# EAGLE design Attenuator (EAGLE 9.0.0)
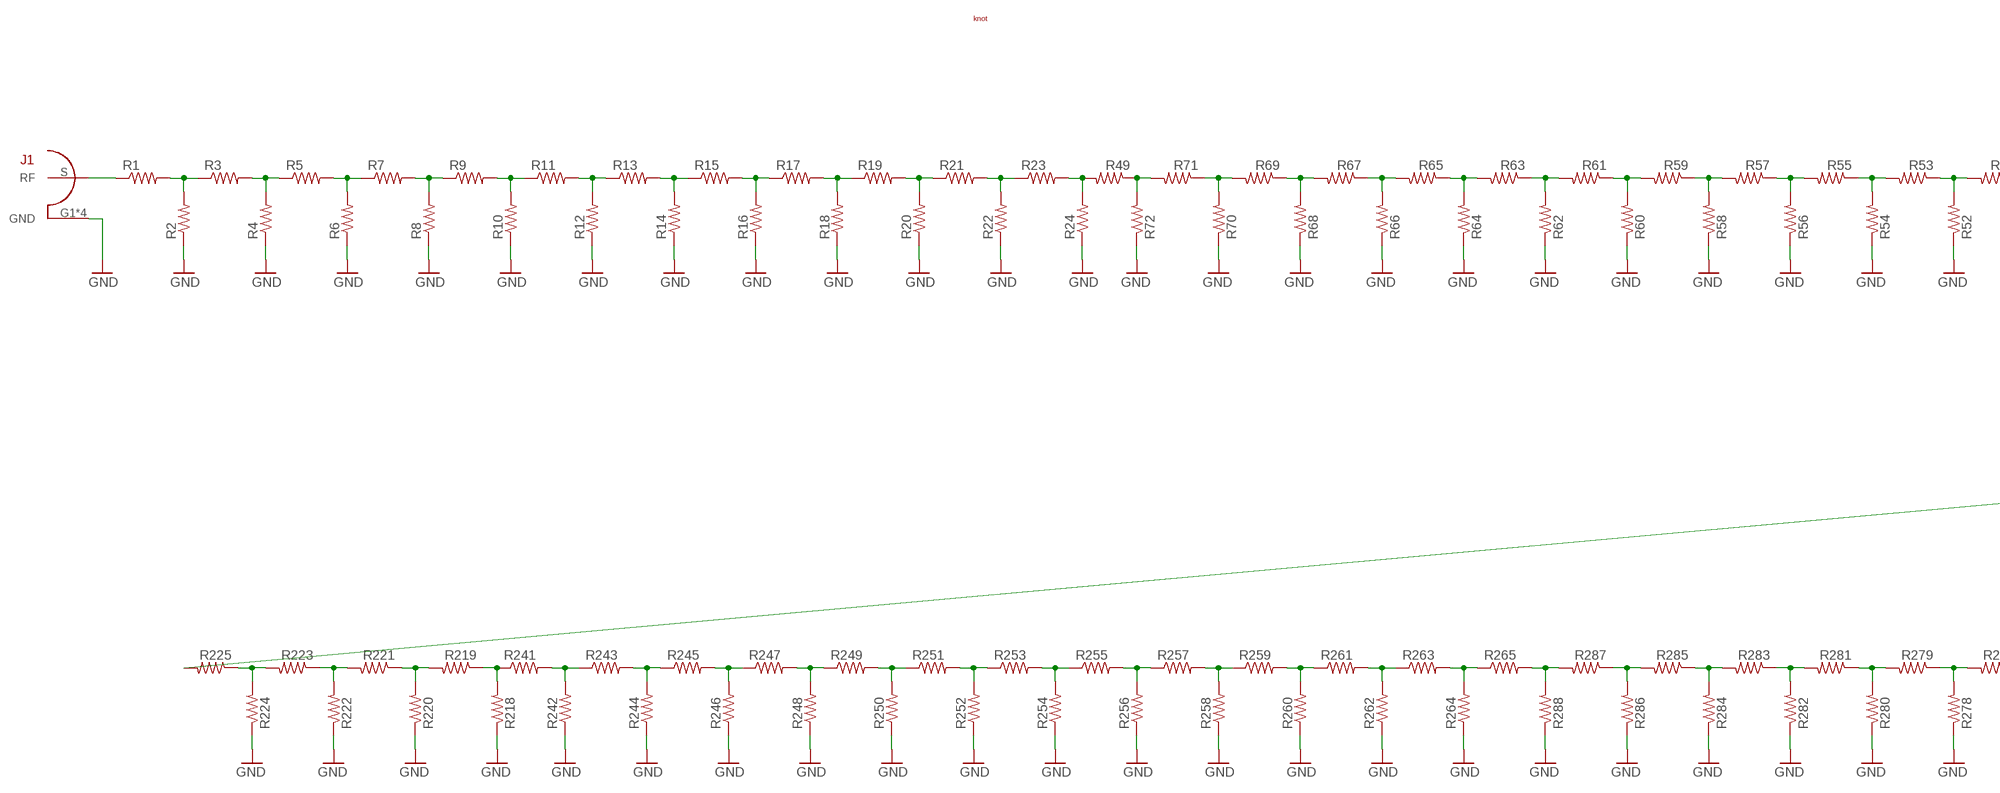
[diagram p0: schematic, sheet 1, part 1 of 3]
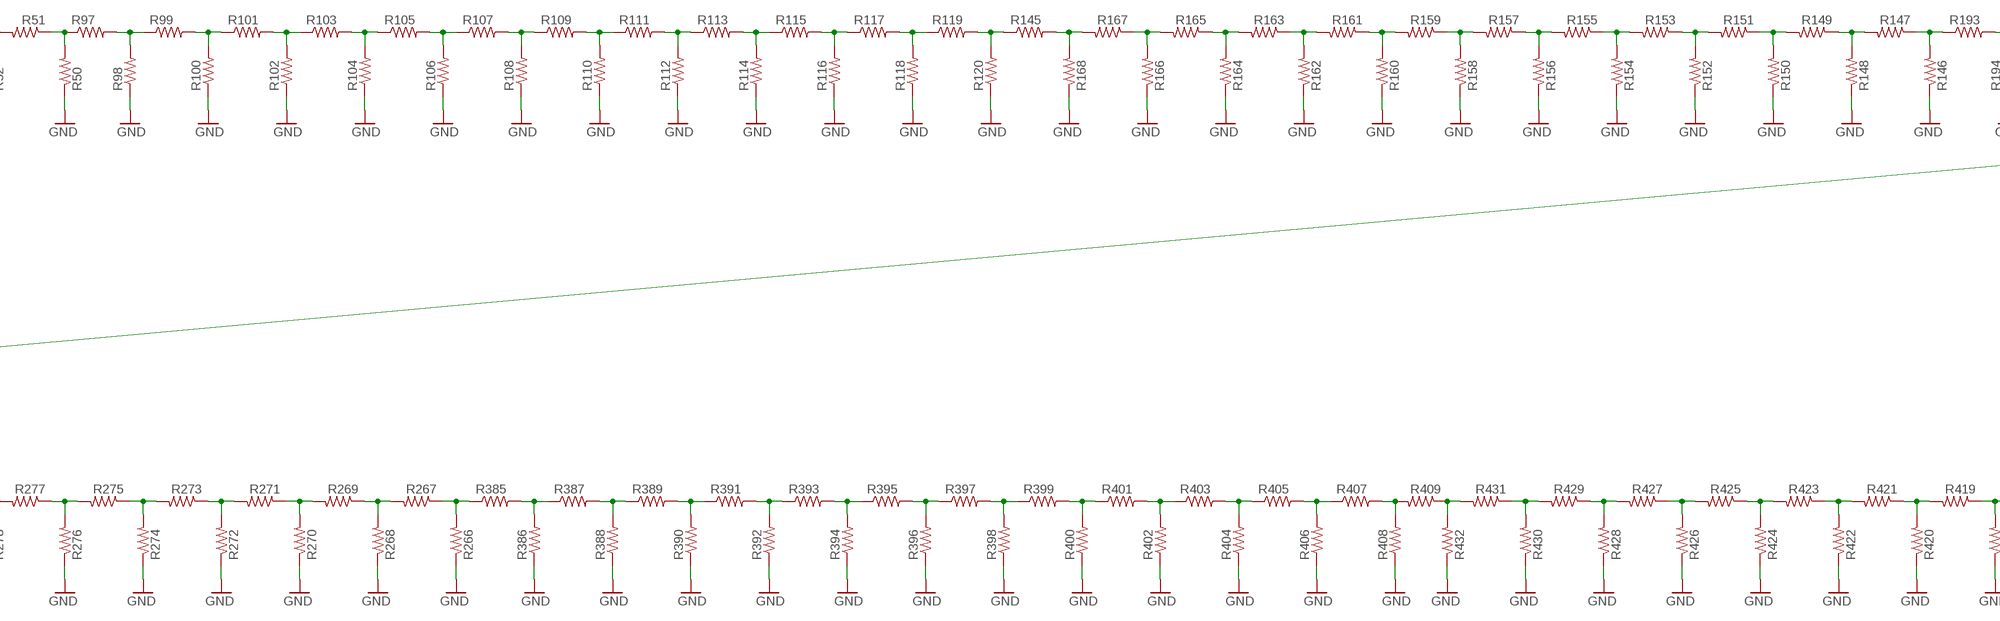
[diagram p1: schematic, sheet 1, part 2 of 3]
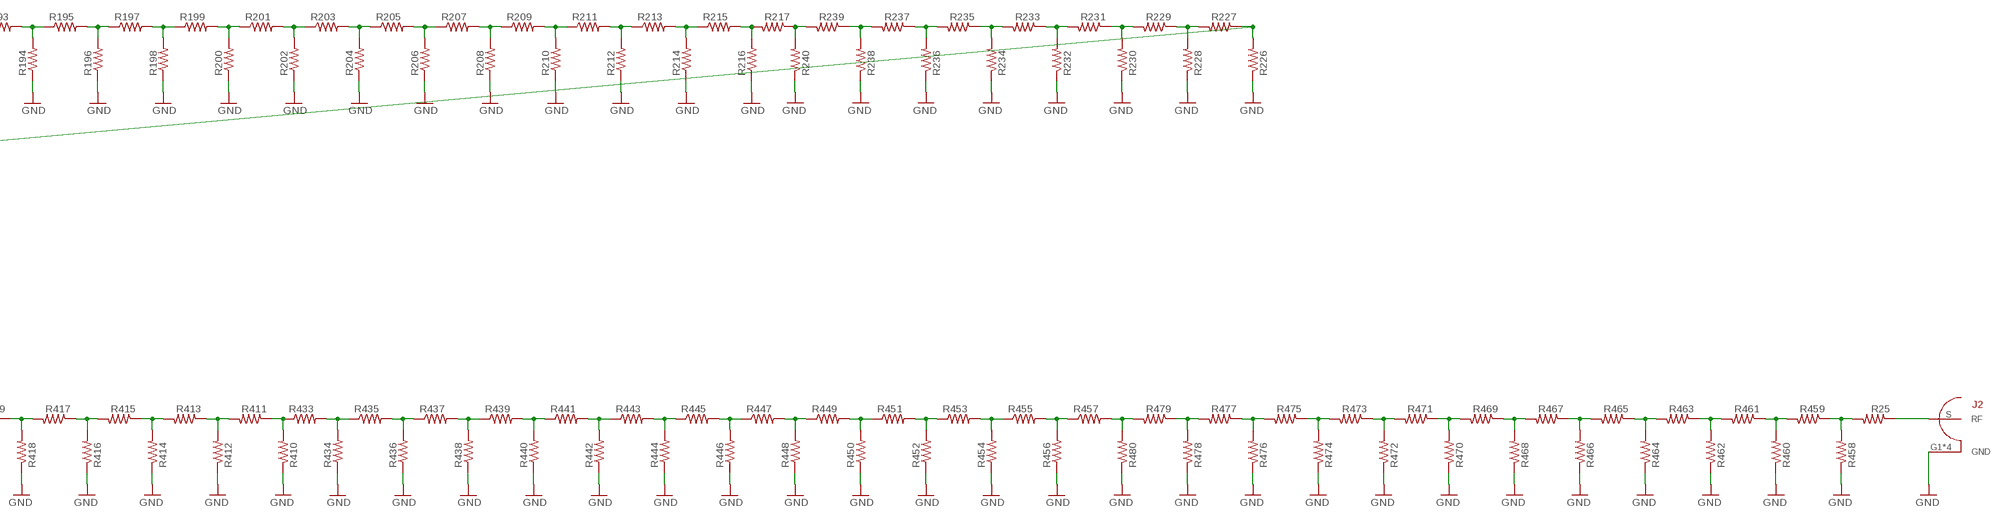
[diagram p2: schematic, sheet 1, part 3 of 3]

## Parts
J1  SMA_0732511150  [WIDE_SMA]
J2  SMA_0732511150  [WIDE_SMA]
R1  R-US_R1206  [R1206]
R2  R-US_R1206  [R1206]
R3  R-US_R1206  [R1206]
R4  R-US_R1206  [R1206]
R5  R-US_R1206  [R1206]
R6  R-US_R1206  [R1206]
R7  R-US_R1206  [R1206]
R8  R-US_R1206  [R1206]
R9  R-US_R1206  [R1206]
R10  R-US_R1206  [R1206]
R11  R-US_R1206  [R1206]
R12  R-US_R1206  [R1206]
R13  R-US_R1206  [R1206]
R14  R-US_R1206  [R1206]
R15  R-US_R1206  [R1206]
R16  R-US_R1206  [R1206]
R17  R-US_R1206  [R1206]
R18  R-US_R1206  [R1206]
R19  R-US_R1206  [R1206]
R20  R-US_R1206  [R1206]
R21  R-US_R1206  [R1206]
R22  R-US_R1206  [R1206]
R23  R-US_R1206  [R1206]
R24  R-US_R1206  [R1206]
R25  R-US_R1206  [R1206]
R49  R-US_R1206  [R1206]
R50  R-US_R1206  [R1206]
R51  R-US_R1206  [R1206]
R52  R-US_R1206  [R1206]
R53  R-US_R1206  [R1206]
R54  R-US_R1206  [R1206]
R55  R-US_R1206  [R1206]
R56  R-US_R1206  [R1206]
R57  R-US_R1206  [R1206]
R58  R-US_R1206  [R1206]
R59  R-US_R1206  [R1206]
R60  R-US_R1206  [R1206]
R61  R-US_R1206  [R1206]
R62  R-US_R1206  [R1206]
R63  R-US_R1206  [R1206]
R64  R-US_R1206  [R1206]
R65  R-US_R1206  [R1206]
R66  R-US_R1206  [R1206]
R67  R-US_R1206  [R1206]
R68  R-US_R1206  [R1206]
R69  R-US_R1206  [R1206]
R70  R-US_R1206  [R1206]
R71  R-US_R1206  [R1206]
R72  R-US_R1206  [R1206]
R97  R-US_R1206  [R1206]
R98  R-US_R1206  [R1206]
R99  R-US_R1206  [R1206]
R100  R-US_R1206  [R1206]
R101  R-US_R1206  [R1206]
R102  R-US_R1206  [R1206]
R103  R-US_R1206  [R1206]
R104  R-US_R1206  [R1206]
R105  R-US_R1206  [R1206]
R106  R-US_R1206  [R1206]
R107  R-US_R1206  [R1206]
R108  R-US_R1206  [R1206]
R109  R-US_R1206  [R1206]
R110  R-US_R1206  [R1206]
R111  R-US_R1206  [R1206]
R112  R-US_R1206  [R1206]
R113  R-US_R1206  [R1206]
R114  R-US_R1206  [R1206]
R115  R-US_R1206  [R1206]
R116  R-US_R1206  [R1206]
R117  R-US_R1206  [R1206]
R118  R-US_R1206  [R1206]
R119  R-US_R1206  [R1206]
R120  R-US_R1206  [R1206]
R145  R-US_R1206  [R1206]
R146  R-US_R1206  [R1206]
R147  R-US_R1206  [R1206]
R148  R-US_R1206  [R1206]
R149  R-US_R1206  [R1206]
R150  R-US_R1206  [R1206]
R151  R-US_R1206  [R1206]
R152  R-US_R1206  [R1206]
R153  R-US_R1206  [R1206]
R154  R-US_R1206  [R1206]
R155  R-US_R1206  [R1206]
R156  R-US_R1206  [R1206]
R157  R-US_R1206  [R1206]
R158  R-US_R1206  [R1206]
R159  R-US_R1206  [R1206]
R160  R-US_R1206  [R1206]
R161  R-US_R1206  [R1206]
R162  R-US_R1206  [R1206]
R163  R-US_R1206  [R1206]
R164  R-US_R1206  [R1206]
R165  R-US_R1206  [R1206]
R166  R-US_R1206  [R1206]
R167  R-US_R1206  [R1206]
R168  R-US_R1206  [R1206]
R193  R-US_R1206  [R1206]
R194  R-US_R1206  [R1206]
R195  R-US_R1206  [R1206]
R196  R-US_R1206  [R1206]
R197  R-US_R1206  [R1206]
R198  R-US_R1206  [R1206]
R199  R-US_R1206  [R1206]
R200  R-US_R1206  [R1206]
R201  R-US_R1206  [R1206]
R202  R-US_R1206  [R1206]
R203  R-US_R1206  [R1206]
R204  R-US_R1206  [R1206]
R205  R-US_R1206  [R1206]
R206  R-US_R1206  [R1206]
R207  R-US_R1206  [R1206]
R208  R-US_R1206  [R1206]
R209  R-US_R1206  [R1206]
R210  R-US_R1206  [R1206]
R211  R-US_R1206  [R1206]
R212  R-US_R1206  [R1206]
R213  R-US_R1206  [R1206]
R214  R-US_R1206  [R1206]
R215  R-US_R1206  [R1206]
R216  R-US_R1206  [R1206]
R217  R-US_R1206  [R1206]
R218  R-US_R1206  [R1206]
R219  R-US_R1206  [R1206]
R220  R-US_R1206  [R1206]
R221  R-US_R1206  [R1206]
R222  R-US_R1206  [R1206]
R223  R-US_R1206  [R1206]
R224  R-US_R1206  [R1206]
R225  R-US_R1206  [R1206]
R226  R-US_R1206  [R1206]
R227  R-US_R1206  [R1206]
R228  R-US_R1206  [R1206]
R229  R-US_R1206  [R1206]
R230  R-US_R1206  [R1206]
R231  R-US_R1206  [R1206]
R232  R-US_R1206  [R1206]
R233  R-US_R1206  [R1206]
R234  R-US_R1206  [R1206]
R235  R-US_R1206  [R1206]
R236  R-US_R1206  [R1206]
R237  R-US_R1206  [R1206]
R238  R-US_R1206  [R1206]
R239  R-US_R1206  [R1206]
R240  R-US_R1206  [R1206]
R241  R-US_R1206  [R1206]
R242  R-US_R1206  [R1206]
R243  R-US_R1206  [R1206]
R244  R-US_R1206  [R1206]
R245  R-US_R1206  [R1206]
R246  R-US_R1206  [R1206]
R247  R-US_R1206  [R1206]
R248  R-US_R1206  [R1206]
R249  R-US_R1206  [R1206]
R250  R-US_R1206  [R1206]
R251  R-US_R1206  [R1206]
R252  R-US_R1206  [R1206]
R253  R-US_R1206  [R1206]
R254  R-US_R1206  [R1206]
R255  R-US_R1206  [R1206]
R256  R-US_R1206  [R1206]
R257  R-US_R1206  [R1206]
R258  R-US_R1206  [R1206]
R259  R-US_R1206  [R1206]
R260  R-US_R1206  [R1206]
R261  R-US_R1206  [R1206]
R262  R-US_R1206  [R1206]
R263  R-US_R1206  [R1206]
R264  R-US_R1206  [R1206]
R265  R-US_R1206  [R1206]
R266  R-US_R1206  [R1206]
R267  R-US_R1206  [R1206]
R268  R-US_R1206  [R1206]
R269  R-US_R1206  [R1206]
R270  R-US_R1206  [R1206]
R271  R-US_R1206  [R1206]
R272  R-US_R1206  [R1206]
R273  R-US_R1206  [R1206]
R274  R-US_R1206  [R1206]
R275  R-US_R1206  [R1206]
R276  R-US_R1206  [R1206]
R277  R-US_R1206  [R1206]
R278  R-US_R1206  [R1206]
R279  R-US_R1206  [R1206]
R280  R-US_R1206  [R1206]
R281  R-US_R1206  [R1206]
R282  R-US_R1206  [R1206]
R283  R-US_R1206  [R1206]
R284  R-US_R1206  [R1206]
R285  R-US_R1206  [R1206]
R286  R-US_R1206  [R1206]
R287  R-US_R1206  [R1206]
R288  R-US_R1206  [R1206]
R385  R-US_R1206  [R1206]
R386  R-US_R1206  [R1206]
R387  R-US_R1206  [R1206]
R388  R-US_R1206  [R1206]
R389  R-US_R1206  [R1206]
R390  R-US_R1206  [R1206]
R391  R-US_R1206  [R1206]
R392  R-US_R1206  [R1206]
R393  R-US_R1206  [R1206]
R394  R-US_R1206  [R1206]
R395  R-US_R1206  [R1206]
R396  R-US_R1206  [R1206]
R397  R-US_R1206  [R1206]
R398  R-US_R1206  [R1206]
R399  R-US_R1206  [R1206]
R400  R-US_R1206  [R1206]
R401  R-US_R1206  [R1206]
R402  R-US_R1206  [R1206]
R403  R-US_R1206  [R1206]
R404  R-US_R1206  [R1206]
R405  R-US_R1206  [R1206]
R406  R-US_R1206  [R1206]
R407  R-US_R1206  [R1206]
R408  R-US_R1206  [R1206]
R409  R-US_R1206  [R1206]
R410  R-US_R1206  [R1206]
R411  R-US_R1206  [R1206]
R412  R-US_R1206  [R1206]
R413  R-US_R1206  [R1206]
R414  R-US_R1206  [R1206]
R415  R-US_R1206  [R1206]
R416  R-US_R1206  [R1206]
R417  R-US_R1206  [R1206]
R418  R-US_R1206  [R1206]
R419  R-US_R1206  [R1206]
R420  R-US_R1206  [R1206]
R421  R-US_R1206  [R1206]
R422  R-US_R1206  [R1206]
R423  R-US_R1206  [R1206]
R424  R-US_R1206  [R1206]
R425  R-US_R1206  [R1206]
R426  R-US_R1206  [R1206]
R427  R-US_R1206  [R1206]
R428  R-US_R1206  [R1206]
R429  R-US_R1206  [R1206]
R430  R-US_R1206  [R1206]
R431  R-US_R1206  [R1206]
R432  R-US_R1206  [R1206]
R433  R-US_R1206  [R1206]
R434  R-US_R1206  [R1206]
R435  R-US_R1206  [R1206]
R436  R-US_R1206  [R1206]
R437  R-US_R1206  [R1206]
R438  R-US_R1206  [R1206]
R439  R-US_R1206  [R1206]
R440  R-US_R1206  [R1206]
R441  R-US_R1206  [R1206]
R442  R-US_R1206  [R1206]
R443  R-US_R1206  [R1206]
R444  R-US_R1206  [R1206]
R445  R-US_R1206  [R1206]
R446  R-US_R1206  [R1206]
R447  R-US_R1206  [R1206]
R448  R-US_R1206  [R1206]
R449  R-US_R1206  [R1206]
R450  R-US_R1206  [R1206]
R451  R-US_R1206  [R1206]
R452  R-US_R1206  [R1206]
R453  R-US_R1206  [R1206]
R454  R-US_R1206  [R1206]
R455  R-US_R1206  [R1206]
R456  R-US_R1206  [R1206]
R457  R-US_R1206  [R1206]
R458  R-US_R1206  [R1206]
R459  R-US_R1206  [R1206]
R460  R-US_R1206  [R1206]
R461  R-US_R1206  [R1206]
R462  R-US_R1206  [R1206]
R463  R-US_R1206  [R1206]
R464  R-US_R1206  [R1206]
R465  R-US_R1206  [R1206]
R466  R-US_R1206  [R1206]
R467  R-US_R1206  [R1206]
R468  R-US_R1206  [R1206]
R469  R-US_R1206  [R1206]
R470  R-US_R1206  [R1206]
R471  R-US_R1206  [R1206]
R472  R-US_R1206  [R1206]
R473  R-US_R1206  [R1206]
R474  R-US_R1206  [R1206]
R475  R-US_R1206  [R1206]
R476  R-US_R1206  [R1206]
R477  R-US_R1206  [R1206]
R478  R-US_R1206  [R1206]
R479  R-US_R1206  [R1206]
R480  R-US_R1206  [R1206]
U$1  THIEF_FULL  [THIEF_KNOT]

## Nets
GND: J1.G1(GND) J1.G2(GND) J1.G3(GND) J1.G4(GND) J2.G1(GND) J2.G2(GND) J2.G3(GND) J2.G4(GND) R2.1 R4.1 R6.1 R8.1 R10.1 R12.1 R14.1 R16.1 R18.1 R20.1 R22.1 R24.1 R50.1 R52.1 R54.1 R56.1 R58.1 R60.1 R62.1 R64.1 R66.1 R68.1 R70.1 R72.1 R98.1 R100.1 R102.1 R104.1 R106.1 R108.1 R110.1 R112.1 R114.1 R116.1 R118.1 R120.1 R146.1 R148.1 R150.1 R152.1 R154.1 R156.1 R158.1 R160.1 R162.1 R164.1 R166.1 R168.1 R194.1 R196.1 R198.1 R200.1 R202.1 R204.1 R206.1 R208.1 R210.1 R212.1 R214.1 R216.1 R218.1 R220.1 R222.1 R224.1 R226.1 R228.1 R230.1 R232.1 R234.1 R236.1 R238.1 R240.1 R242.1 R244.1 R246.1 R248.1 R250.1 R252.1 R254.1 R256.1 R258.1 R260.1 R262.1 R264.1 R266.1 R268.1 R270.1 R272.1 R274.1 R276.1 R278.1 R280.1 R282.1 R284.1 R286.1 R288.1 R386.1 R388.1 R390.1 R392.1 R394.1 R396.1 R398.1 R400.1 R402.1 R404.1 R406.1 R408.1 R410.1 R412.1 R414.1 R416.1 R418.1 R420.1 R422.1 R424.1 R426.1 R428.1 R430.1 R432.1 R434.1 R436.1 R438.1 R440.1 R442.1 R444.1 R446.1 R448.1 R450.1 R452.1 R454.1 R456.1 R458.1 R460.1 R462.1 R464.1 R466.1 R468.1 R470.1 R472.1 R474.1 R476.1 R478.1 R480.1
N$1: R1.2 R2.2 R3.1
N$2: R3.2 R4.2 R5.1
N$3: R5.2 R6.2 R7.1
N$4: R7.2 R8.2 R9.1
N$5: R9.2 R10.2 R11.1
N$6: R11.2 R12.2 R13.1
N$7: R13.2 R14.2 R15.1
N$8: R15.2 R16.2 R17.1
N$9: R17.2 R18.2 R19.1
N$10: R19.2 R20.2 R21.1
N$11: R21.2 R22.2 R23.1
N$12: R23.2 R24.2 R49.2
N$13: J1.S(RF) R1.1
N$14: J2.S(RF) R25.1
N$25: R50.2 R51.1 R97.1
N$26: R51.2 R52.2 R53.1
N$27: R53.2 R54.2 R55.1
N$28: R55.2 R56.2 R57.1
N$29: R57.2 R58.2 R59.1
N$30: R59.2 R60.2 R61.1
N$31: R61.2 R62.2 R63.1
N$32: R63.2 R64.2 R65.1
N$33: R65.2 R66.2 R67.1
N$34: R67.2 R68.2 R69.1
N$35: R69.2 R70.2 R71.1
N$36: R49.1 R71.2 R72.2
N$49: R97.2 R98.2 R99.1
N$50: R99.2 R100.2 R101.1
N$51: R101.2 R102.2 R103.1
N$52: R103.2 R104.2 R105.1
N$53: R105.2 R106.2 R107.1
N$54: R107.2 R108.2 R109.1
N$55: R109.2 R110.2 R111.1
N$56: R111.2 R112.2 R113.1
N$57: R113.2 R114.2 R115.1
N$58: R115.2 R116.2 R117.1
N$59: R117.2 R118.2 R119.1
N$60: R119.2 R120.2 R145.1
N$73: R146.2 R147.1 R193.1
N$74: R147.2 R148.2 R149.1
N$75: R149.2 R150.2 R151.1
N$76: R151.2 R152.2 R153.1
N$77: R153.2 R154.2 R155.1
N$78: R155.2 R156.2 R157.1
N$79: R157.2 R158.2 R159.1
N$80: R159.2 R160.2 R161.1
N$81: R161.2 R162.2 R163.1
N$82: R163.2 R164.2 R165.1
N$83: R165.2 R166.2 R167.1
N$84: R145.2 R167.2 R168.2
N$97: R193.2 R194.2 R195.1
N$98: R195.2 R196.2 R197.1
N$99: R197.2 R198.2 R199.1
N$100: R199.2 R200.2 R201.1
N$101: R201.2 R202.2 R203.1
N$102: R203.2 R204.2 R205.1
N$103: R205.2 R206.2 R207.1
N$104: R207.2 R208.2 R209.1
N$105: R209.2 R210.2 R211.1
N$106: R211.2 R212.2 R213.1
N$107: R213.2 R214.2 R215.1
N$108: R215.2 R216.2 R217.2
N$109: R218.2 R219.1 R241.1
N$110: R219.2 R220.2 R221.1
N$111: R221.2 R222.2 R223.1
N$112: R223.2 R224.2 R225.1
N$113: R225.2 R226.2 R227.1
N$114: R227.2 R228.2 R229.1
N$115: R229.2 R230.2 R231.1
N$116: R231.2 R232.2 R233.1
N$117: R233.2 R234.2 R235.1
N$118: R235.2 R236.2 R237.1
N$119: R237.2 R238.2 R239.1
N$120: R217.1 R239.2 R240.2
N$121: R241.2 R242.2 R243.1
N$122: R243.2 R244.2 R245.1
N$123: R245.2 R246.2 R247.1
N$124: R247.2 R248.2 R249.1
N$125: R249.2 R250.2 R251.1
N$126: R251.2 R252.2 R253.1
N$127: R253.2 R254.2 R255.1
N$128: R255.2 R256.2 R257.1
N$129: R257.2 R258.2 R259.1
N$130: R259.2 R260.2 R261.1
N$131: R261.2 R262.2 R263.1
N$132: R263.2 R264.2 R265.1
N$133: R266.2 R267.1 R385.1
N$134: R267.2 R268.2 R269.1
N$135: R269.2 R270.2 R271.1
N$136: R271.2 R272.2 R273.1
N$137: R273.2 R274.2 R275.1
N$138: R275.2 R276.2 R277.1
N$139: R277.2 R278.2 R279.1
N$140: R279.2 R280.2 R281.1
N$141: R281.2 R282.2 R283.1
N$142: R283.2 R284.2 R285.1
N$143: R285.2 R286.2 R287.1
N$144: R265.2 R287.2 R288.2
N$193: R385.2 R386.2 R387.1
N$194: R387.2 R388.2 R389.1
N$195: R389.2 R390.2 R391.1
N$196: R391.2 R392.2 R393.1
N$197: R393.2 R394.2 R395.1
N$198: R395.2 R396.2 R397.1
N$199: R397.2 R398.2 R399.1
N$200: R399.2 R400.2 R401.1
N$201: R401.2 R402.2 R403.1
N$202: R403.2 R404.2 R405.1
N$203: R405.2 R406.2 R407.1
N$204: R407.2 R408.2 R409.2
N$205: R410.2 R411.1 R433.1
N$206: R411.2 R412.2 R413.1
N$207: R413.2 R414.2 R415.1
N$208: R415.2 R416.2 R417.1
N$209: R417.2 R418.2 R419.1
N$210: R419.2 R420.2 R421.1
N$211: R421.2 R422.2 R423.1
N$212: R423.2 R424.2 R425.1
N$213: R425.2 R426.2 R427.1
N$214: R427.2 R428.2 R429.1
N$215: R429.2 R430.2 R431.1
N$216: R409.1 R431.2 R432.2
N$217: R433.2 R434.2 R435.1
N$218: R435.2 R436.2 R437.1
N$219: R437.2 R438.2 R439.1
N$220: R439.2 R440.2 R441.1
N$221: R441.2 R442.2 R443.1
N$222: R443.2 R444.2 R445.1
N$223: R445.2 R446.2 R447.1
N$224: R447.2 R448.2 R449.1
N$225: R449.2 R450.2 R451.1
N$226: R451.2 R452.2 R453.1
N$227: R453.2 R454.2 R455.1
N$228: R455.2 R456.2 R457.1
N$229: R25.2 R458.2 R459.1
N$230: R459.2 R460.2 R461.1
N$231: R461.2 R462.2 R463.1
N$232: R463.2 R464.2 R465.1
N$233: R465.2 R466.2 R467.1
N$234: R467.2 R468.2 R469.1
N$235: R469.2 R470.2 R471.1
N$236: R471.2 R472.2 R473.1
N$237: R473.2 R474.2 R475.1
N$238: R475.2 R476.2 R477.1
N$239: R477.2 R478.2 R479.1
N$240: R457.2 R479.2 R480.2

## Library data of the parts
J1 J2 = ruark2:SMA_0732511150: SMA Connector Receptacle, Female Socket 50 Ohm Board Edge, End Launch Solder; PARTNO: WM5534-ND
R1-R25 R49-R72 R97-R120 R145-R168 R193-R288 R385-R480 = resistor:R-US_: RESISTOR, American symbol
U$1 = ruark2:THIEF_FULL; PARTNO: NA

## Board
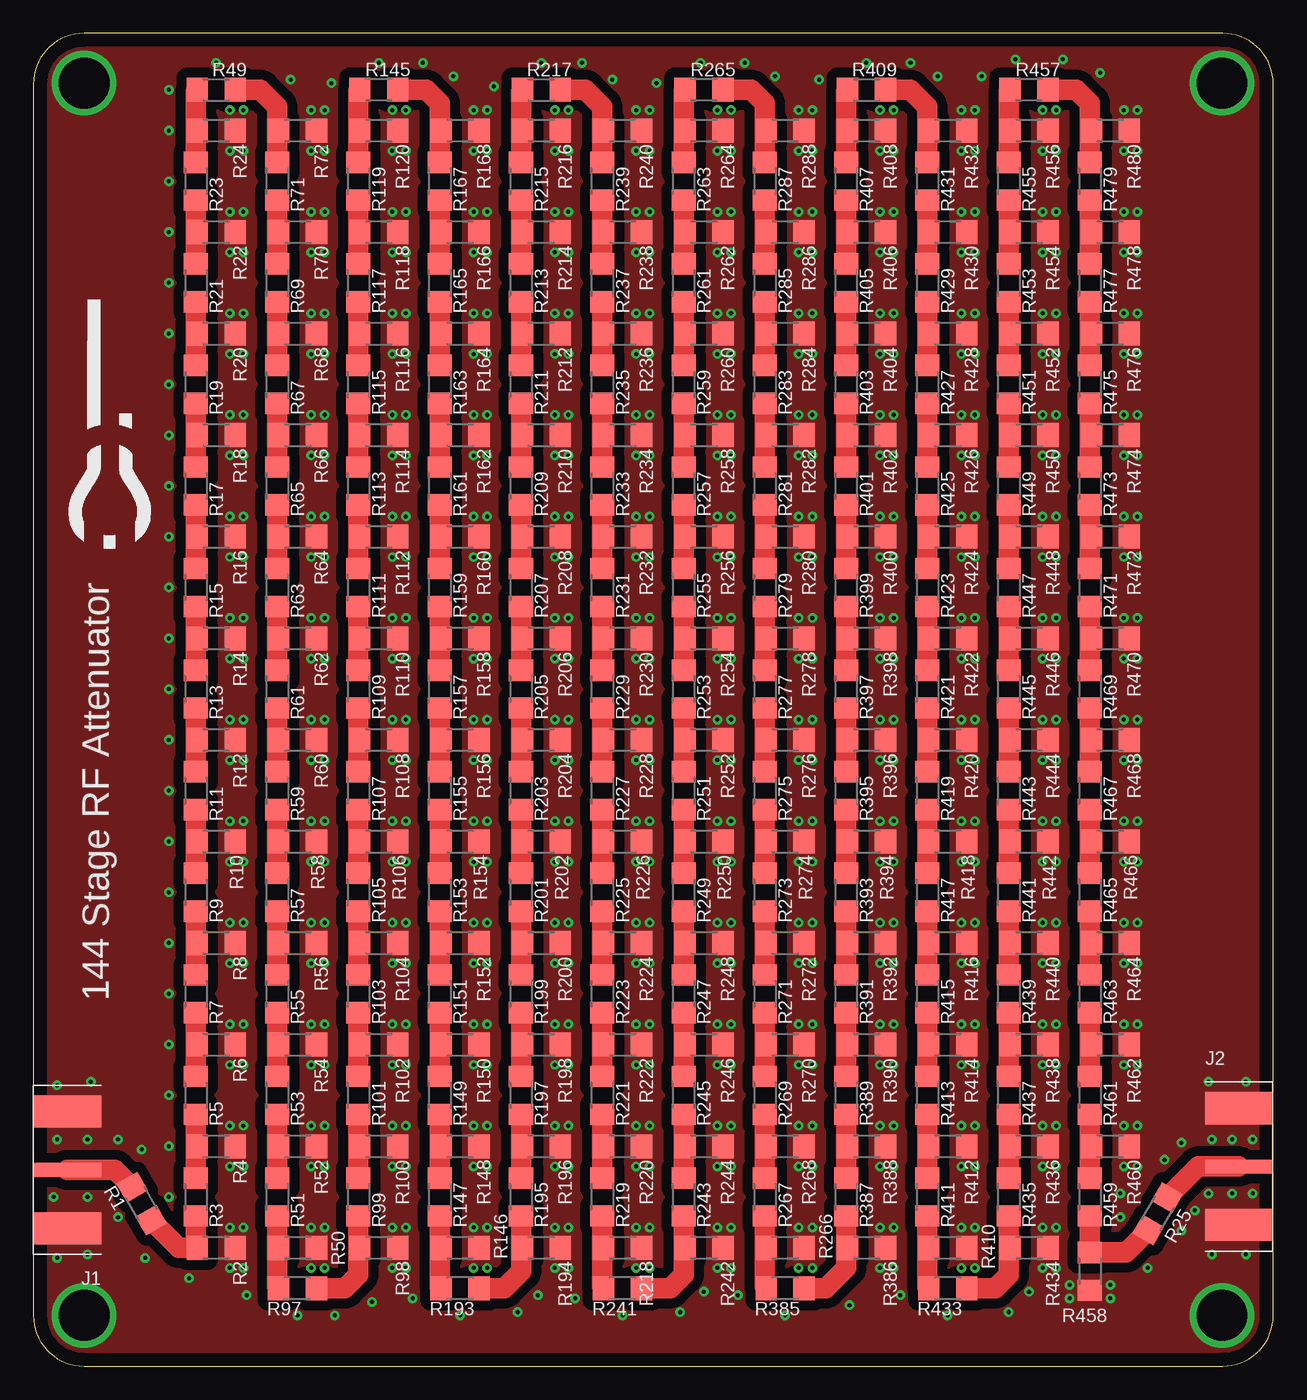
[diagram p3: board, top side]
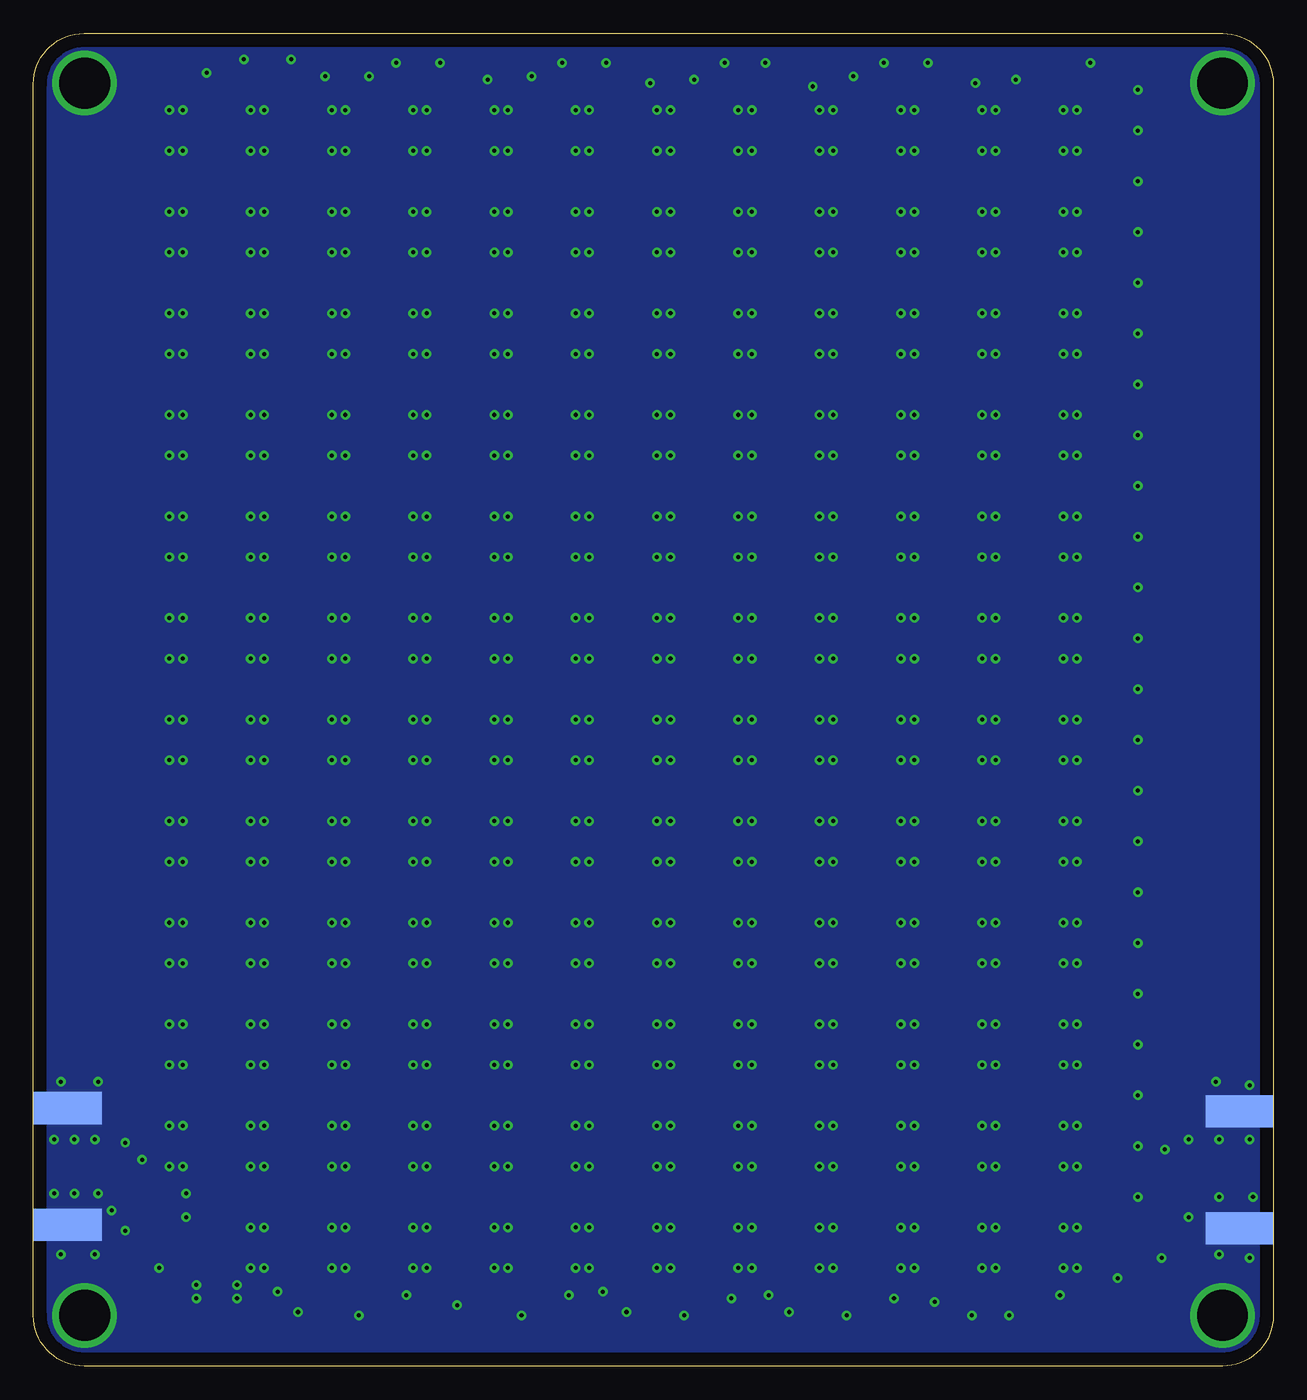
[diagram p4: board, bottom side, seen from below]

Size 93 x 100 mm. Coordinates in mm from the lower left corner, seen from the top.
Outline: 3.81,0 89.19,0 arc90 93,3.81 93,96.19 arc90 89.19,100 3.81,100 arc90 0,96.19 0,3.81 arc90 3.81,0
Copper layers (1*16): Top 0.035mm / dielectric 1.5mm / Bottom 0.035mm
Design rules "default": minimum track width 6mil, minimum drill 0.35mm, track to track 6mil, track to pad 6mil, pad to pad 6mil, via to via 6mil, smd to smd 6mil, copper to edge 40mil, drill to drill 6mil, minimum pad ring 10mil, minimum via ring 8mil, stop-mask expansion 4mil, vias tented up to drill 0mil, thermal gap 10mil

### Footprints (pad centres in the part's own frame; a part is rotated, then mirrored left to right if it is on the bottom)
WIDE_SMA = smd 5.08 x 2.413 bottom: G1 0,4.381; G4 0,-4.381 | smd 5.08 x 2.413: G2 0,-4.381; G3 0,4.381 | smd 5.08 x 1.016: S 0,0
R1206 = smd 1.6 x 1.803: 1 -1.422,0; 2 1.422,0

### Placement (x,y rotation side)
J1  2.54,14.73 180 top
J2  90.42,14.99 0 top
R1  8.13,12.19 300 top
R2  13.72,8.89 180 top
R3  12.19,12.7 90 top
R4  13.72,16.51 180 top
R5  12.19,20.32 90 top
R6  13.72,24.13 180 top
R7  12.19,27.94 90 top
R8  13.72,31.75 180 top
R9  12.19,35.56 90 top
R10  13.72,39.37 180 top
R11  12.19,43.18 90 top
R12  13.72,46.99 180 top
R13  12.19,50.8 90 top
R14  13.72,54.61 180 top
R15  12.19,58.42 90 top
R16  13.72,62.23 180 top
R17  12.19,66.04 90 top
R18  13.72,69.85 180 top
R19  12.19,73.66 90 top
R20  13.72,77.47 180 top
R21  12.19,81.28 90 top
R22  13.72,85.09 180 top
R23  12.19,88.9 90 top
R24  13.72,92.71 180 top
R25  84.33,11.43 240 top
R49  13.72,95.76 180 top
R50  19.81,8.89 180 top
R51  18.29,12.7 90 top
R52  19.81,16.51 180 top
R53  18.29,20.32 90 top
R54  19.81,24.13 180 top
R55  18.29,27.94 90 top
R56  19.81,31.75 180 top
R57  18.29,35.56 90 top
R58  19.81,39.37 180 top
R59  18.29,43.18 90 top
R60  19.81,46.99 180 top
R61  18.29,50.8 90 top
R62  19.81,54.61 180 top
R63  18.29,58.42 90 top
R64  19.81,62.23 180 top
R65  18.29,66.04 90 top
R66  19.81,69.85 180 top
R67  18.29,73.66 90 top
R68  19.81,77.47 180 top
R69  18.29,81.28 90 top
R70  19.81,85.09 180 top
R71  18.29,88.9 90 top
R72  19.81,92.71 180 top
R97  19.81,5.84 0 top
R98  25.91,8.89 180 top
R99  24.38,12.7 90 top
R100  25.91,16.51 180 top
R101  24.38,20.32 90 top
R102  25.91,24.13 180 top
R103  24.38,27.94 90 top
R104  25.91,31.75 180 top
R105  24.38,35.56 90 top
R106  25.91,39.37 180 top
R107  24.38,43.18 90 top
R108  25.91,46.99 180 top
R109  24.38,50.8 90 top
R110  25.91,54.61 180 top
R111  24.38,58.42 90 top
R112  25.91,62.23 180 top
R113  24.38,66.04 90 top
R114  25.91,69.85 180 top
R115  24.38,73.66 90 top
R116  25.91,77.47 180 top
R117  24.38,81.28 90 top
R118  25.91,85.09 180 top
R119  24.38,88.9 90 top
R120  25.91,92.71 180 top
R145  25.91,95.76 0 top
R146  32,8.89 180 top
R147  30.48,12.7 90 top
R148  32,16.51 180 top
R149  30.48,20.32 90 top
R150  32,24.13 180 top
R151  30.48,27.94 90 top
R152  32,31.75 180 top
R153  30.48,35.56 90 top
R154  32,39.37 180 top
R155  30.48,43.18 90 top
R156  32,46.99 180 top
R157  30.48,50.8 90 top
R158  32,54.61 180 top
R159  30.48,58.42 90 top
R160  32,62.23 180 top
R161  30.48,66.04 90 top
R162  32,69.85 180 top
R163  30.48,73.66 90 top
R164  32,77.47 180 top
R165  30.48,81.28 90 top
R166  32,85.09 180 top
R167  30.48,88.9 90 top
R168  32,92.71 180 top
R193  32,5.84 0 top
R194  38.1,8.89 180 top
R195  36.58,12.7 90 top
R196  38.1,16.51 180 top
R197  36.58,20.32 90 top
R198  38.1,24.13 180 top
R199  36.58,27.94 90 top
R200  38.1,31.75 180 top
R201  36.58,35.56 90 top
R202  38.1,39.37 180 top
R203  36.58,43.18 90 top
R204  38.1,46.99 180 top
R205  36.58,50.8 90 top
R206  38.1,54.61 180 top
R207  36.58,58.42 90 top
R208  38.1,62.23 180 top
R209  36.58,66.04 90 top
R210  38.1,69.85 180 top
R211  36.58,73.66 90 top
R212  38.1,77.47 180 top
R213  36.58,81.28 90 top
R214  38.1,85.09 180 top
R215  36.58,88.9 90 top
R216  38.1,92.71 180 top
R217  38.1,95.76 180 top
R218  44.2,8.89 180 top
R219  42.67,12.7 90 top
R220  44.2,16.51 180 top
R221  42.67,20.32 90 top
R222  44.2,24.13 180 top
R223  42.67,27.94 90 top
R224  44.2,31.75 180 top
R225  42.67,35.56 90 top
R226  44.2,39.37 180 top
R227  42.67,43.18 90 top
R228  44.2,46.99 180 top
R229  42.67,50.8 90 top
R230  44.2,54.61 180 top
R231  42.67,58.42 90 top
R232  44.2,62.23 180 top
R233  42.67,66.04 90 top
R234  44.2,69.85 180 top
R235  42.67,73.66 90 top
R236  44.2,77.47 180 top
R237  42.67,81.28 90 top
R238  44.2,85.09 180 top
R239  42.67,88.9 90 top
R240  44.2,92.71 180 top
R241  44.2,5.84 0 top
R242  50.29,8.89 180 top
R243  48.77,12.7 90 top
R244  50.29,16.51 180 top
R245  48.77,20.32 90 top
R246  50.29,24.13 180 top
R247  48.77,27.94 90 top
R248  50.29,31.75 180 top
R249  48.77,35.56 90 top
R250  50.29,39.37 180 top
R251  48.77,43.18 90 top
R252  50.29,46.99 180 top
R253  48.77,50.8 90 top
R254  50.29,54.61 180 top
R255  48.77,58.42 90 top
R256  50.29,62.23 180 top
R257  48.77,66.04 90 top
R258  50.29,69.85 180 top
R259  48.77,73.66 90 top
R260  50.29,77.47 180 top
R261  48.77,81.28 90 top
R262  50.29,85.09 180 top
R263  48.77,88.9 90 top
R264  50.29,92.71 180 top
R265  50.29,95.76 0 top
R266  56.39,8.89 180 top
R267  54.86,12.7 90 top
R268  56.39,16.51 180 top
R269  54.86,20.32 90 top
R270  56.39,24.13 180 top
R271  54.86,27.94 90 top
R272  56.39,31.75 180 top
R273  54.86,35.56 90 top
R274  56.39,39.37 180 top
R275  54.86,43.18 90 top
R276  56.39,46.99 180 top
R277  54.86,50.8 90 top
R278  56.39,54.61 180 top
R279  54.86,58.42 90 top
R280  56.39,62.23 180 top
R281  54.86,66.04 90 top
R282  56.39,69.85 180 top
R283  54.86,73.66 90 top
R284  56.39,77.47 180 top
R285  54.86,81.28 90 top
R286  56.39,85.09 180 top
R287  54.86,88.9 90 top
R288  56.39,92.71 180 top
R385  56.39,5.84 0 top
R386  62.48,8.89 180 top
R387  60.96,12.7 90 top
R388  62.48,16.51 180 top
R389  60.96,20.32 90 top
R390  62.48,24.13 180 top
R391  60.96,27.94 90 top
R392  62.48,31.75 180 top
R393  60.96,35.56 90 top
R394  62.48,39.37 180 top
R395  60.96,43.18 90 top
R396  62.48,46.99 180 top
R397  60.96,50.8 90 top
R398  62.48,54.61 180 top
R399  60.96,58.42 90 top
R400  62.48,62.23 180 top
R401  60.96,66.04 90 top
R402  62.48,69.85 180 top
R403  60.96,73.66 90 top
R404  62.48,77.47 180 top
R405  60.96,81.28 90 top
R406  62.48,85.09 180 top
R407  60.96,88.9 90 top
R408  62.48,92.71 180 top
R409  62.48,95.76 180 top
R410  68.58,8.89 180 top
R411  67.06,12.7 90 top
R412  68.58,16.51 180 top
R413  67.06,20.32 90 top
R414  68.58,24.13 180 top
R415  67.06,27.94 90 top
R416  68.58,31.75 180 top
R417  67.06,35.56 90 top
R418  68.58,39.37 180 top
R419  67.06,43.18 90 top
R420  68.58,46.99 180 top
R421  67.06,50.8 90 top
R422  68.58,54.61 180 top
R423  67.06,58.42 90 top
R424  68.58,62.23 180 top
R425  67.06,66.04 90 top
R426  68.58,69.85 180 top
R427  67.06,73.66 90 top
R428  68.58,77.47 180 top
R429  67.06,81.28 90 top
R430  68.58,85.09 180 top
R431  67.06,88.9 90 top
R432  68.58,92.71 180 top
R433  68.58,5.84 0 top
R434  74.68,8.89 180 top
R435  73.15,12.7 90 top
R436  74.68,16.51 180 top
R437  73.15,20.32 90 top
R438  74.68,24.13 180 top
R439  73.15,27.94 90 top
R440  74.68,31.75 180 top
R441  73.15,35.56 90 top
R442  74.68,39.37 180 top
R443  73.15,43.18 90 top
R444  74.68,46.99 180 top
R445  73.15,50.8 90 top
R446  74.68,54.61 180 top
R447  73.15,58.42 90 top
R448  74.68,62.23 180 top
R449  73.15,66.04 90 top
R450  74.68,69.85 180 top
R451  73.15,73.66 90 top
R452  74.68,77.47 180 top
R453  73.15,81.28 90 top
R454  74.68,85.09 180 top
R455  73.15,88.9 90 top
R456  74.68,92.71 180 top
R457  74.68,95.76 0 top
R458  79.25,7.11 90 top
R459  79.25,12.7 90 top
R460  80.77,16.51 180 top
R461  79.25,20.32 90 top
R462  80.77,24.13 180 top
R463  79.25,27.94 90 top
R464  80.77,31.75 180 top
R465  79.25,35.56 90 top
R466  80.77,39.37 180 top
R467  79.25,43.18 90 top
R468  80.77,46.99 180 top
R469  79.25,50.8 90 top
R470  80.77,54.61 180 top
R471  79.25,58.42 90 top
R472  80.77,62.23 180 top
R473  79.25,66.04 90 top
R474  80.77,69.85 180 top
R475  79.25,73.66 90 top
R476  80.77,77.47 180 top
R477  79.25,81.28 90 top
R478  80.77,85.09 180 top
R479  79.25,88.9 90 top
R480  80.77,92.71 180 top
U$1  1.02,77.72 270 top

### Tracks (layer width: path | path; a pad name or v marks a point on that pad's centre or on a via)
GND  (via drill 0.3, 3.81)
  other vias: 14.73,10.41 15.75,10.41 15.75,7.37 14.73,7.37 14.73,14.99 15.75,14.99 14.73,18.03 15.75,18.03 14.73,22.61 15.75,22.61 14.73,25.65 15.75,25.65 14.73,30.23 15.75,30.23 14.73,33.27 15.75,33.27 14.73,37.85 15.75,37.85 14.73,40.89 15.75,40.89 14.73,45.47 15.75,45.47 14.73,48.51 15.75,48.51 14.73,53.09 15.75,53.09 14.73,56.13 15.75,56.13 14.73,60.71 15.75,60.71 14.73,63.75 15.75,63.75 14.73,68.33 15.75,68.33 14.73,71.37 15.75,71.37 14.73,75.95 15.75,75.95 14.73,78.99 15.75,78.99 14.73,83.57 15.75,83.57 14.73,86.61 15.75,86.61 14.73,91.19 15.75,91.19 14.73,94.23 15.75,94.23 20.83,10.41 21.84,10.41 21.84,7.37 20.83,7.37 20.83,14.99 21.84,14.99 20.83,18.03 21.84,18.03 20.83,22.61 21.84,22.61 20.83,25.65 21.84,25.65 20.83,30.23 21.84,30.23 20.83,33.27 21.84,33.27 20.83,37.85 21.84,37.85 20.83,40.89 21.84,40.89 20.83,45.47 21.84,45.47 20.83,48.51 21.84,48.51 20.83,53.09 21.84,53.09 20.83,56.13 21.84,56.13 20.83,60.71 21.84,60.71 20.83,63.75 21.84,63.75 20.83,68.33 21.84,68.33 20.83,71.37 21.84,71.37 20.83,75.95 21.84,75.95 20.83,78.99 21.84,78.99 20.83,83.57 21.84,83.57 20.83,86.61 21.84,86.61 20.83,91.19 21.84,91.19 20.83,94.23 21.84,94.23 26.92,10.41 27.94,10.41 27.94,7.37 26.92,7.37 26.92,14.99 27.94,14.99 26.92,18.03 27.94,18.03 26.92,22.61 27.94,22.61 26.92,25.65 27.94,25.65 26.92,30.23 27.94,30.23 26.92,33.27 27.94,33.27 26.92,37.85 27.94,37.85 26.92,40.89 27.94,40.89 26.92,45.47 27.94,45.47 26.92,48.51 27.94,48.51 26.92,53.09 27.94,53.09 26.92,56.13 27.94,56.13 26.92,60.71 27.94,60.71 26.92,63.75 27.94,63.75 26.92,68.33 27.94,68.33 26.92,71.37 27.94,71.37 26.92,75.95 27.94,75.95 26.92,78.99 27.94,78.99 26.92,83.57 27.94,83.57 26.92,86.61 27.94,86.61 26.92,91.19 27.94,91.19 26.92,94.23 27.94,94.23 33.02,10.41 34.04,10.41 34.04,7.37 33.02,7.37 33.02,14.99 34.04,14.99 33.02,18.03 34.04,18.03 33.02,22.61 34.04,22.61 33.02,25.65 34.04,25.65 33.02,30.23 34.04,30.23 33.02,33.27 34.04,33.27 33.02,37.85 34.04,37.85 33.02,40.89 34.04,40.89 33.02,45.47 34.04,45.47 33.02,48.51 34.04,48.51 33.02,53.09 34.04,53.09 33.02,56.13 34.04,56.13 33.02,60.71 34.04,60.71 33.02,63.75 34.04,63.75 33.02,68.33 34.04,68.33 33.02,71.37 34.04,71.37 33.02,75.95 34.04,75.95 33.02,78.99 34.04,78.99 33.02,83.57 34.04,83.57 33.02,86.61 34.04,86.61 33.02,91.19 34.04,91.19 33.02,94.23 34.04,94.23 39.12,10.41 40.13,10.41 40.13,7.37 39.12,7.37 39.12,14.99 40.13,14.99 39.12,18.03 40.13,18.03 39.12,22.61 40.13,22.61 39.12,25.65 40.13,25.65 39.12,30.23 40.13,30.23 39.12,33.27 40.13,33.27 39.12,37.85 40.13,37.85 39.12,40.89 40.13,40.89 39.12,45.47 40.13,45.47 39.12,48.51 40.13,48.51 39.12,53.09 40.13,53.09 39.12,56.13 40.13,56.13 39.12,60.71 40.13,60.71 39.12,63.75 40.13,63.75 39.12,68.33 40.13,68.33 39.12,71.37 40.13,71.37 39.12,75.95 40.13,75.95 39.12,78.99 40.13,78.99 39.12,83.57 40.13,83.57 39.12,86.61 40.13,86.61 39.12,91.19 40.13,91.19 39.12,94.23 40.13,94.23 45.21,10.41 46.23,10.41 46.23,7.37 45.21,7.37 45.21,14.99 46.23,14.99 45.21,18.03 46.23,18.03 45.21,22.61 46.23,22.61 45.21,25.65 46.23,25.65 45.21,30.23 46.23,30.23 45.21,33.27 46.23,33.27 45.21,37.85 46.23,37.85 45.21,40.89 46.23,40.89 45.21,45.47 46.23,45.47 45.21,48.51 46.23,48.51 45.21,53.09 46.23,53.09 45.21,56.13 46.23,56.13 45.21,60.71 46.23,60.71 45.21,63.75 46.23,63.75 45.21,68.33 46.23,68.33 45.21,71.37 46.23,71.37 45.21,75.95 46.23,75.95 45.21,78.99 46.23,78.99 45.21,83.57 46.23,83.57 45.21,86.61 46.23,86.61 45.21,91.19 46.23,91.19 45.21,94.23 46.23,94.23 51.31,10.41 52.32,10.41 52.32,7.37 51.31,7.37 51.31,14.99 52.32,14.99 51.31,18.03 52.32,18.03 51.31,22.61 52.32,22.61 51.31,25.65 52.32,25.65 51.31,30.23 52.32,30.23 51.31,33.27 52.32,33.27 51.31,37.85 52.32,37.85 51.31,40.89 52.32,40.89 51.31,45.47 52.32,45.47 51.31,48.51 52.32,48.51 51.31,53.09 52.32,53.09 51.31,56.13 52.32,56.13 51.31,60.71 52.32,60.71 51.31,63.75 52.32,63.75 51.31,68.33 52.32,68.33 51.31,71.37 52.32,71.37 51.31,75.95 52.32,75.95 51.31,78.99 52.32,78.99 51.31,83.57 52.32,83.57 51.31,86.61 52.32,86.61 51.31,91.19 52.32,91.19 51.31,94.23 52.32,94.23 57.4,10.41 58.42,10.41 58.42,7.37 57.4,7.37 57.4,14.99 58.42,14.99 57.4,18.03 58.42,18.03 57.4,22.61 58.42,22.61 57.4,25.65 58.42,25.65 57.4,30.23 58.42,30.23 57.4,33.27 58.42,33.27 57.4,37.85 58.42,37.85 57.4,40.89 58.42,40.89 57.4,45.47 58.42,45.47 57.4,48.51 58.42,48.51 57.4,53.09 58.42,53.09 57.4,56.13 58.42,56.13 57.4,60.71 58.42,60.71 57.4,63.75 58.42,63.75 57.4,68.33 58.42,68.33 57.4,71.37 58.42,71.37 57.4,75.95 58.42,75.95 57.4,78.99 58.42,78.99 57.4,83.57 58.42,83.57 57.4,86.61 58.42,86.61 57.4,91.19 58.42,91.19 57.4,94.23 58.42,94.23 63.5,10.41 64.52,10.41 64.52,7.37 63.5,7.37 63.5,14.99 64.52,14.99 63.5,18.03 64.52,18.03 63.5,22.61 64.52,22.61 63.5,25.65 64.52,25.65 63.5,30.23 64.52,30.23 63.5,33.27 64.52,33.27 63.5,37.85 64.52,37.85 63.5,40.89 64.52,40.89 63.5,45.47 64.52,45.47 63.5,48.51 64.52,48.51 63.5,53.09 64.52,53.09 63.5,56.13 64.52,56.13 63.5,60.71 64.52,60.71 63.5,63.75 64.52,63.75 63.5,68.33 64.52,68.33 63.5,71.37 64.52,71.37 63.5,75.95 64.52,75.95 63.5,78.99 64.52,78.99 63.5,83.57 64.52,83.57 63.5,86.61 64.52,86.61 63.5,91.19 64.52,91.19 63.5,94.23 64.52,94.23 69.6,10.41 70.61,10.41 70.61,7.37 69.6,7.37 69.6,14.99 70.61,14.99 69.6,18.03 70.61,18.03 69.6,22.61 70.61,22.61 69.6,25.65 70.61,25.65 69.6,30.23 70.61,30.23 69.6,33.27 70.61,33.27 69.6,37.85 70.61,37.85 69.6,40.89 70.61,40.89 69.6,45.47 70.61,45.47 69.6,48.51 70.61,48.51 69.6,53.09 70.61,53.09 69.6,56.13 70.61,56.13 69.6,60.71 70.61,60.71 69.6,63.75 70.61,63.75 69.6,68.33 70.61,68.33 69.6,71.37 70.61,71.37 69.6,75.95 70.61,75.95 69.6,78.99 70.61,78.99 69.6,83.57 70.61,83.57 69.6,86.61 70.61,86.61 69.6,91.19 70.61,91.19 69.6,94.23 70.61,94.23 75.69,10.41 76.71,10.41 76.71,7.37 75.69,7.37 75.69,14.99 76.71,14.99 75.69,18.03 76.71,18.03 75.69,22.61 76.71,22.61 75.69,25.65 76.71,25.65 75.69,30.23 76.71,30.23 75.69,33.27 76.71,33.27 75.69,37.85 76.71,37.85 75.69,40.89 76.71,40.89 75.69,45.47 76.71,45.47 75.69,48.51 76.71,48.51 75.69,53.09 76.71,53.09 75.69,56.13 76.71,56.13 75.69,60.71 76.71,60.71 75.69,63.75 76.71,63.75 75.69,68.33 76.71,68.33 75.69,71.37 76.71,71.37 75.69,75.95 76.71,75.95 75.69,78.99 76.71,78.99 75.69,83.57 76.71,83.57 75.69,86.61 76.71,86.61 75.69,91.19 76.71,91.19 75.69,94.23 76.71,94.23 80.77,6.1 80.77,5.08 77.72,5.08 77.72,6.1 81.79,14.99 82.8,14.99 81.79,18.03 82.8,18.03 81.79,22.61 82.8,22.61 81.79,25.65 82.8,25.65 81.79,30.23 82.8,30.23 81.79,33.27 82.8,33.27 81.79,37.85 82.8,37.85 81.79,40.89 82.8,40.89 81.79,45.47 82.8,45.47 81.79,48.51 82.8,48.51 81.79,53.09 82.8,53.09 81.79,56.13 82.8,56.13 81.79,60.71 82.8,60.71 81.79,63.75 82.8,63.75 81.79,68.33 82.8,68.33 81.79,71.37 82.8,71.37 81.79,75.95 82.8,75.95 81.79,78.99 82.8,78.99 81.79,83.57 82.8,83.57 81.79,86.61 82.8,86.61 81.79,91.19 82.8,91.19 81.79,94.23 82.8,94.23 3.81,3.81 89.15,3.81 89.15,96.27 3.81,96.27 19.3,96.52 13.72,97.79 10.16,95.76 10.16,88.9 10.16,92.71 10.16,85.09 10.16,81.28 10.16,77.47 10.16,73.66 10.16,69.85 10.16,66.04 10.16,62.23 10.16,58.42 10.16,54.61 10.16,50.8 10.16,46.99 10.16,43.18 10.16,39.37 10.16,35.56 10.16,31.75 10.16,27.94 10.16,24.13 10.16,20.32 10.16,16.51 10.16,12.7 8.13,16.26 4.06,17.02 6.35,11.18 8.38,8.13 11.68,6.6 16,5.33 19.81,3.81 22.61,3.81 25.4,4.83 28.45,5.08 32,3.81 36.32,4.06 37.85,5.33 40.64,5.08 44.2,3.81 48.51,4.06 50.29,5.59 52.83,5.33 56.39,3.81 61.21,4.57 65.02,5.33 68.58,3.81 73.15,4.06 74.68,5.59 83.57,7.37 86.11,10.16 88.14,12.95 81.53,11.18 81.53,12.95 84.84,15.49 88.39,17.02 22.35,96.27 25.91,97.79 29.21,97.79 31.5,96.77 34.54,96.01 38.1,97.79 41.15,97.79 43.43,96.52 46.74,96.27 50.04,97.79 53.34,97.79 55.63,96.77 58.93,96.52 62.48,97.79 65.79,97.79 67.82,96.77 71.12,96.77 73.66,98.04 77.22,98.04 80.01,97.03 1.78,17.02 6.35,17.02 4.06,12.7 1.52,12.7 86.11,16.76 89.92,17.02 91.44,17.02 89.92,12.95 91.44,12.95 87.12,11.68 1.78,8.13 4.06,8.38 1.78,21.08 4.32,21.34 90.93,8.38 88.39,8.38 90.93,21.34 88.14,21.34
  pour Bottom (no thermals): -2.54,104.14 106.68,104.14 106.68,-2.54 -7.62,-2.54 -7.62,104.14
  pour Top (isolate 0.762, no thermals): 0,100.84 93.22,100.84 93.22,-0.25 -0.25,-0.25 -0.25,100.84
N$1
  Top 1.524: 12.19,8.89 R3.1 | R2.2 12.19,8.89 | R1.2 10.91,8.89 12.19,8.89
N$2
  Top 1.524: R3.2 12.19,16.51 | 12.19,16.51 R5.1 | R4.2 12.19,16.51
N$3
  Top 1.524: R5.2 12.19,24.13 | 12.19,24.13 R7.1 | R6.2 12.19,24.13
N$4
  Top 1.524: R7.2 12.19,31.75 | 12.19,31.75 R9.1 | R8.2 12.19,31.75
N$5
  Top 1.524: R9.2 12.19,39.37 | 12.19,39.37 R11.1 | R10.2 12.19,39.37
N$6
  Top 1.524: R11.2 12.19,46.99 | 12.19,46.99 R13.1 | R12.2 12.19,46.99
N$7
  Top 1.524: R13.2 12.19,54.61 | 12.19,54.61 R15.1 | R14.2 12.19,54.61
N$8
  Top 1.524: R15.2 12.19,62.13 | 12.19,62.13 R17.1 | R16.2 12.19,62.13
N$9
  Top 1.524: R17.2 12.19,69.75 | 12.19,69.75 R19.1 | R18.2 12.19,69.75
N$10
  Top 1.524: R19.2 12.19,77.47 | 12.19,77.47 R21.1 | R20.2 12.19,77.47
N$11
  Top 1.524: R21.2 12.19,85.09 | 12.19,85.09 R23.1 | R22.2 12.19,85.09
N$12
  Top 1.524: R24.2 12.19,92.61 R23.2 12.19,95.66 R49.2
N$13
  Top 1.524: R1.1 6.11,14.73 J1.S
N$14
  Top 1.524: R25.1 87.36,14.99 J2.S
N$25
  Top 1.524: 18.29,8.89 R51.1 | R50.2 18.29,8.89 | R97.1 18.29,5.94 18.29,8.89
N$26
  Top 1.524: R51.2 18.29,16.51 | 18.29,16.51 R53.1 | R52.2 18.29,16.51
N$27
  Top 1.524: R53.2 18.29,24.13 | 18.29,24.13 R55.1 | R54.2 18.29,24.13
N$28
  Top 1.524: R55.2 18.29,31.75 | 18.29,31.75 R57.1 | R56.2 18.29,31.75
N$29
  Top 1.524: R57.2 18.29,39.37 | 18.29,39.37 R59.1 | R58.2 18.29,39.37
N$30
  Top 1.524: R59.2 18.29,46.99 | 18.29,46.99 R61.1 | R60.2 18.29,46.99
N$31
  Top 1.524: R61.2 18.29,54.61 | 18.29,54.61 R63.1 | R62.2 18.29,54.61
N$32
  Top 1.524: R63.2 18.29,62.13 | 18.29,62.13 R65.1 | R64.2 18.29,62.13
N$33
  Top 1.524: R65.2 18.29,69.75 | 18.29,69.75 R67.1 | R66.2 18.29,69.75
N$34
  Top 1.524: R67.2 18.29,77.47 | 18.29,77.47 R69.1 | R68.2 18.29,77.47
N$35
  Top 1.524: R69.2 18.29,85.09 | 18.29,85.09 R71.1 | R70.2 18.29,85.09
N$36
  Top 1.524: R71.2 18.29,92.61 | 18.29,92.61 R72.2 | R49.1 17.02,95.76 18.29,94.49 18.29,92.61
N$49
  Top 1.524: 24.38,8.89 R99.1 | R98.2 24.38,8.89 | R97.2 23.37,5.84 24.38,6.86 24.38,8.89
N$50
  Top 1.524: R99.2 24.38,16.51 | 24.38,16.51 R101.1 | R100.2 24.38,16.51
N$51
  Top 1.524: R101.2 24.38,24.13 | 24.38,24.13 R103.1 | R102.2 24.38,24.13
N$52
  Top 1.524: R103.2 24.38,31.75 | 24.38,31.75 R105.1 | R104.2 24.38,31.75
N$53
  Top 1.524: R105.2 24.38,39.37 | 24.38,39.37 R107.1 | R106.2 24.38,39.37
N$54
  Top 1.524: R107.2 24.38,46.99 | 24.38,46.99 R109.1 | R108.2 24.38,46.99
N$55
  Top 1.524: R109.2 24.38,54.61 | 24.38,54.61 R111.1 | R110.2 24.38,54.61
N$56
  Top 1.524: R111.2 24.38,62.13 | 24.38,62.13 R113.1 | R112.2 24.38,62.13
N$57
  Top 1.524: R113.2 24.38,69.75 | 24.38,69.75 R115.1 | R114.2 24.38,69.75
N$58
  Top 1.524: R115.2 24.38,77.47 | 24.38,77.47 R117.1 | R116.2 24.38,77.47
N$59
  Top 1.524: R117.2 24.38,85.09 | 24.38,85.09 R119.1 | R118.2 24.38,85.09
N$60
  Top 1.524: R120.2 24.38,92.61 R119.2 24.38,95.66 R145.1
N$73
  Top 1.524: 30.48,8.89 R147.1 | R146.2 30.48,8.89 | R193.1 30.48,5.94 30.48,8.89
N$74
  Top 1.524: R147.2 30.48,16.51 | 30.48,16.51 R149.1 | R148.2 30.48,16.51
N$75
  Top 1.524: R149.2 30.48,24.13 | 30.48,24.13 R151.1 | R150.2 30.48,24.13
N$76
  Top 1.524: R151.2 30.48,31.75 | 30.48,31.75 R153.1 | R152.2 30.48,31.75
N$77
  Top 1.524: R153.2 30.48,39.37 | 30.48,39.37 R155.1 | R154.2 30.48,39.37
N$78
  Top 1.524: R155.2 30.48,46.99 | 30.48,46.99 R157.1 | R156.2 30.48,46.99
N$79
  Top 1.524: R157.2 30.48,54.61 | 30.48,54.61 R159.1 | R158.2 30.48,54.61
N$80
  Top 1.524: R159.2 30.48,62.13 | 30.48,62.13 R161.1 | R160.2 30.48,62.13
N$81
  Top 1.524: R161.2 30.48,69.75 | 30.48,69.75 R163.1 | R162.2 30.48,69.75
N$82
  Top 1.524: R163.2 30.48,77.47 | 30.48,77.47 R165.1 | R164.2 30.48,77.47
N$83
  Top 1.524: R165.2 30.48,85.09 | 30.48,85.09 R167.1 | R166.2 30.48,85.09
N$84
  Top 1.524: R168.2 30.48,92.61 R167.2 30.48,94.74 29.46,95.76 R145.2
N$97
  Top 1.524: 36.58,8.89 R195.1 | R194.2 36.58,8.89 | R193.2 35.31,5.84 36.58,7.11 36.58,8.89
N$98
  Top 1.524: R195.2 36.58,16.51 | 36.58,16.51 R197.1 | R196.2 36.58,16.51
N$99
  Top 1.524: R197.2 36.58,24.13 | 36.58,24.13 R199.1 | R198.2 36.58,24.13
N$100
  Top 1.524: R199.2 36.58,31.75 | 36.58,31.75 R201.1 | R200.2 36.58,31.75
N$101
  Top 1.524: R201.2 36.58,39.37 | 36.58,39.37 R203.1 | R202.2 36.58,39.37
N$102
  Top 1.524: R203.2 36.58,46.99 | 36.58,46.99 R205.1 | R204.2 36.58,46.99
N$103
  Top 1.524: R205.2 36.58,54.61 | 36.58,54.61 R207.1 | R206.2 36.58,54.61
N$104
  Top 1.524: R207.2 36.58,62.13 | 36.58,62.13 R209.1 | R208.2 36.58,62.13
N$105
  Top 1.524: R209.2 36.58,69.75 | 36.58,69.75 R211.1 | R210.2 36.58,69.75
N$106
  Top 1.524: R211.2 36.58,77.47 | 36.58,77.47 R213.1 | R212.2 36.58,77.47
N$107
  Top 1.524: R213.2 36.58,85.09 | 36.58,85.09 R215.1 | R214.2 36.58,85.09
N$108
  Top 1.524: R216.2 36.58,92.61 R215.2 36.58,95.66 R217.2
N$109
  Top 1.524: 42.67,8.89 R219.1 | R218.2 42.67,8.89 | R241.1 42.67,5.94 42.67,8.89
N$110
  Top 1.524: R219.2 42.67,16.51 | 42.67,16.51 R221.1 | R220.2 42.67,16.51
N$111
  Top 1.524: R221.2 42.67,24.13 | 42.67,24.13 R223.1 | R222.2 42.67,24.13
N$112
  Top 1.524: R223.2 42.67,31.75 | 42.67,31.75 R225.1 | R224.2 42.67,31.75
N$113
  Top 1.524: R225.2 42.67,39.37 | 42.67,39.37 R227.1 | R226.2 42.67,39.37
N$114
  Top 1.524: R227.2 42.67,46.99 | 42.67,46.99 R229.1 | R228.2 42.67,46.99
N$115
  Top 1.524: R229.2 42.67,54.61 | 42.67,54.61 R231.1 | R230.2 42.67,54.61
N$116
  Top 1.524: R231.2 42.67,62.13 | 42.67,62.13 R233.1 | R232.2 42.67,62.13
N$117
  Top 1.524: R233.2 42.67,69.75 | 42.67,69.75 R235.1 | R234.2 42.67,69.75
N$118
  Top 1.524: R235.2 42.67,77.47 | 42.67,77.47 R237.1 | R236.2 42.67,77.47
N$119
  Top 1.524: R237.2 42.67,85.09 | 42.67,85.09 R239.1 | R238.2 42.67,85.09
N$120
  Top 1.524: R239.2 42.67,92.61 | 42.67,92.61 R240.2 | R217.1 41.4,95.76 42.67,94.49 42.67,92.61
N$121
  Top 1.524: 48.77,8.89 R243.1 | R242.2 48.77,8.89 | R241.2 47.75,5.84 48.77,6.86 48.77,8.89
N$122
  Top 1.524: R243.2 48.77,16.51 | 48.77,16.51 R245.1 | R244.2 48.77,16.51
N$123
  Top 1.524: R245.2 48.77,24.13 | 48.77,24.13 R247.1 | R246.2 48.77,24.13
N$124
  Top 1.524: R247.2 48.77,31.75 | 48.77,31.75 R249.1 | R248.2 48.77,31.75
N$125
  Top 1.524: R249.2 48.77,39.37 | 48.77,39.37 R251.1 | R250.2 48.77,39.37
N$126
  Top 1.524: R251.2 48.77,46.99 | 48.77,46.99 R253.1 | R252.2 48.77,46.99
N$127
  Top 1.524: R253.2 48.77,54.61 | 48.77,54.61 R255.1 | R254.2 48.77,54.61
N$128
  Top 1.524: R255.2 48.77,62.13 | 48.77,62.13 R257.1 | R256.2 48.77,62.13
N$129
  Top 1.524: R257.2 48.77,69.75 | 48.77,69.75 R259.1 | R258.2 48.77,69.75
N$130
  Top 1.524: R259.2 48.77,77.47 | 48.77,77.47 R261.1 | R260.2 48.77,77.47
N$131
  Top 1.524: R261.2 48.77,85.09 | 48.77,85.09 R263.1 | R262.2 48.77,85.09
N$132
  Top 1.524: R264.2 48.77,92.61 R263.2 48.77,95.66 R265.1
N$133
  Top 1.524: 54.86,8.89 R267.1 | R266.2 54.86,8.89 | R385.1 54.86,5.94 54.86,8.89
N$134
  Top 1.524: R267.2 54.86,16.51 | 54.86,16.51 R269.1 | R268.2 54.86,16.51
N$135
  Top 1.524: R269.2 54.86,24.13 | 54.86,24.13 R271.1 | R270.2 54.86,24.13
N$136
  Top 1.524: R271.2 54.86,31.75 | 54.86,31.75 R273.1 | R272.2 54.86,31.75
N$137
  Top 1.524: R273.2 54.86,39.37 | 54.86,39.37 R275.1 | R274.2 54.86,39.37
N$138
  Top 1.524: R275.2 54.86,46.99 | 54.86,46.99 R277.1 | R276.2 54.86,46.99
N$139
  Top 1.524: R277.2 54.86,54.61 | 54.86,54.61 R279.1 | R278.2 54.86,54.61
N$140
  Top 1.524: R279.2 54.86,62.13 | 54.86,62.13 R281.1 | R280.2 54.86,62.13
N$141
  Top 1.524: R281.2 54.86,69.75 | 54.86,69.75 R283.1 | R282.2 54.86,69.75
N$142
  Top 1.524: R283.2 54.86,77.47 | 54.86,77.47 R285.1 | R284.2 54.86,77.47
N$143
  Top 1.524: R285.2 54.86,85.09 | 54.86,85.09 R287.1 | R286.2 54.86,85.09
N$144
  Top 1.524: R288.2 54.86,92.61 R287.2 54.86,94.74 53.85,95.76 R265.2
N$193
  Top 1.524: 60.96,8.89 R387.1 | R386.2 60.96,8.89 | R385.2 59.44,5.84 60.96,7.37 60.96,8.89
N$194
  Top 1.524: R387.2 60.96,16.51 | 60.96,16.51 R389.1 | R388.2 60.96,16.51
N$195
  Top 1.524: R389.2 60.96,24.13 | 60.96,24.13 R391.1 | R390.2 60.96,24.13
N$196
  Top 1.524: R391.2 60.96,31.75 | 60.96,31.75 R393.1 | R392.2 60.96,31.75
N$197
  Top 1.524: R393.2 60.96,39.37 | 60.96,39.37 R395.1 | R394.2 60.96,39.37
N$198
  Top 1.524: R395.2 60.96,46.99 | 60.96,46.99 R397.1 | R396.2 60.96,46.99
N$199
  Top 1.524: R397.2 60.96,54.61 | 60.96,54.61 R399.1 | R398.2 60.96,54.61
N$200
  Top 1.524: R399.2 60.96,62.13 | 60.96,62.13 R401.1 | R400.2 60.96,62.13
N$201
  Top 1.524: R401.2 60.96,69.75 | 60.96,69.75 R403.1 | R402.2 60.96,69.75
N$202
  Top 1.524: R403.2 60.96,77.47 | 60.96,77.47 R405.1 | R404.2 60.96,77.47
N$203
  Top 1.524: R405.2 60.96,85.09 | 60.96,85.09 R407.1 | R406.2 60.96,85.09
N$204
  Top 1.524: R408.2 60.96,92.61 R407.2 60.96,95.66 R409.2
N$205
  Top 1.524: 67.06,8.89 R411.1 | R410.2 67.06,8.89 | R433.1 67.06,5.94 67.06,8.89
N$206
  Top 1.524: R411.2 67.06,16.51 | 67.06,16.51 R413.1 | R412.2 67.06,16.51
N$207
  Top 1.524: R413.2 67.06,24.13 | 67.06,24.13 R415.1 | R414.2 67.06,24.13
N$208
  Top 1.524: R415.2 67.06,31.75 | 67.06,31.75 R417.1 | R416.2 67.06,31.75
N$209
  Top 1.524: R417.2 67.06,39.37 | 67.06,39.37 R419.1 | R418.2 67.06,39.37
N$210
  Top 1.524: R419.2 67.06,46.99 | 67.06,46.99 R421.1 | R420.2 67.06,46.99
N$211
  Top 1.524: R421.2 67.06,54.61 | 67.06,54.61 R423.1 | R422.2 67.06,54.61
N$212
  Top 1.524: R423.2 67.06,62.13 | 67.06,62.13 R425.1 | R424.2 67.06,62.13
N$213
  Top 1.524: R425.2 67.06,69.75 | 67.06,69.75 R427.1 | R426.2 67.06,69.75
N$214
  Top 1.524: R427.2 67.06,77.47 | 67.06,77.47 R429.1 | R428.2 67.06,77.47
N$215
  Top 1.524: R429.2 67.06,85.09 | 67.06,85.09 R431.1 | R430.2 67.06,85.09
N$216
  Top 1.524: R431.2 67.06,92.61 | 67.06,92.61 R432.2 | R409.1 65.79,95.76 67.06,94.49 67.06,92.61
N$217
  Top 1.524: 73.15,8.89 R435.1 | R434.2 73.15,8.89 | R433.2 72.14,5.84 73.15,6.86 73.15,8.89
N$218
  Top 1.524: R435.2 73.15,16.51 | 73.15,16.51 R437.1 | R436.2 73.15,16.51
N$219
  Top 1.524: R437.2 73.15,24.13 | 73.15,24.13 R439.1 | R438.2 73.15,24.13
N$220
  Top 1.524: R439.2 73.15,31.75 | 73.15,31.75 R441.1 | R440.2 73.15,31.75
N$221
  Top 1.524: R441.2 73.15,39.37 | 73.15,39.37 R443.1 | R442.2 73.15,39.37
N$222
  Top 1.524: R443.2 73.15,46.99 | 73.15,46.99 R445.1 | R444.2 73.15,46.99
N$223
  Top 1.524: R445.2 73.15,54.61 | 73.15,54.61 R447.1 | R446.2 73.15,54.61
N$224
  Top 1.524: R447.2 73.15,62.13 | 73.15,62.13 R449.1 | R448.2 73.15,62.13
N$225
  Top 1.524: R449.2 73.15,69.75 | 73.15,69.75 R451.1 | R450.2 73.15,69.75
N$226
  Top 1.524: R451.2 73.15,77.47 | 73.15,77.47 R453.1 | R452.2 73.15,77.47
N$227
  Top 1.524: R453.2 73.15,85.09 | 73.15,85.09 R455.1 | R454.2 73.15,85.09
N$228
  Top 1.524: R456.2 73.15,92.61 R455.2 73.15,95.66 R457.1
N$229
  Top 1.524: R459.1 R458.2 81.95,8.53 R25.2
N$230
  Top 1.524: R459.2 79.25,16.51 | 79.25,16.51 R461.1 | R460.2 79.25,16.51
N$231
  Top 1.524: R461.2 79.25,24.13 | 79.25,24.13 R463.1 | R462.2 79.25,24.13
N$232
  Top 1.524: R463.2 79.25,31.75 | 79.25,31.75 R465.1 | R464.2 79.25,31.75
N$233
  Top 1.524: R465.2 79.25,39.37 | 79.25,39.37 R467.1 | R466.2 79.25,39.37
N$234
  Top 1.524: R467.2 79.25,46.99 | 79.25,46.99 R469.1 | R468.2 79.25,46.99
N$235
  Top 1.524: R469.2 79.25,54.61 | 79.25,54.61 R471.1 | R470.2 79.25,54.61
N$236
  Top 1.524: R471.2 79.25,62.13 | 79.25,62.13 R473.1 | R472.2 79.25,62.13
N$237
  Top 1.524: R473.2 79.25,69.75 | 79.25,69.75 R475.1 | R474.2 79.25,69.75
N$238
  Top 1.524: R475.2 79.25,77.47 | 79.25,77.47 R477.1 | R476.2 79.25,77.47
N$239
  Top 1.524: R477.2 79.25,85.09 | 79.25,85.09 R479.1 | R478.2 79.25,85.09
N$240
  Top 1.524: R480.2 79.25,92.61 R479.2 79.25,94.74 78.23,95.76 R457.2

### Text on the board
tPlace: 144 Stage RF Attenuator
tStop: MMXX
